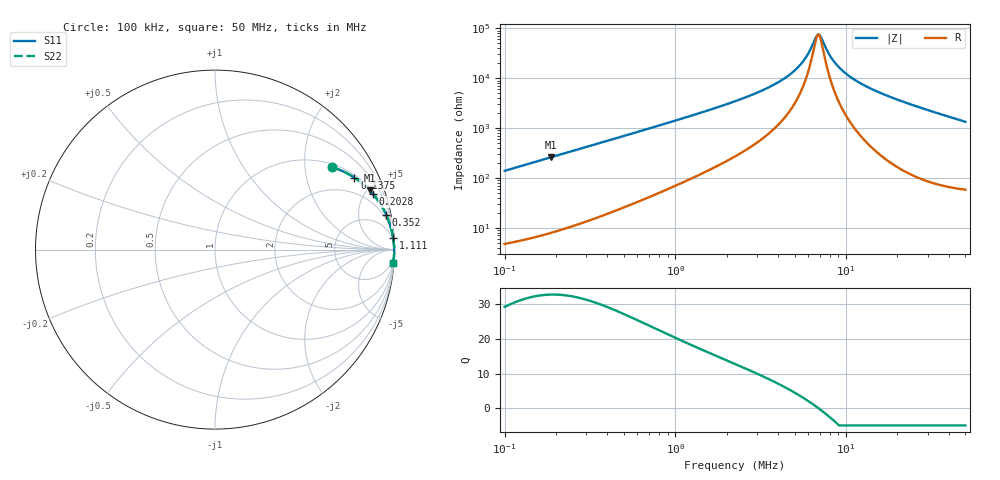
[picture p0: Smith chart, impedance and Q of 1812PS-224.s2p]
# MHz S MA R 50
!Freq  MagS11  AngS11  MagS21  AngS21  MagS12  AngS12  MagS22  AngS22
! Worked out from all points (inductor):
!   801 points, 100 kHz to 50 MHz, reference 50 ohm
!   read as one part in series: L = 220 uH near 103.2 kHz
!   highest Q = 32.8 at 186.2 kHz (marker M1), where L = 220 uH
!   self-resonance near 6.844 MHz
!   S11 on the Smith chart (normalised r, x): 100 kHz: 1.09, +2.76; 137.5 kHz: 1.12, +3.80; 202.8 kHz: 1.17, +5.61; 352 kHz: 1.32, +9.75; 1.111 MHz: 3, +31; 50 MHz: 2, -27
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0.1  0.7976 35.2  0.5766 -52.9  0.5766 -52.9  0.7976 35.2
0.1375062  0.8739 27.3  0.4595 -60.9  0.4595 -60.9  0.8739 27.3
0.1861646  0.9228 21.0  0.3583 -67.3  0.3583 -67.3  0.9228 21.0
0.2027719  0.933 19.4  0.3326 -68.8  0.3326 -68.8  0.933 19.4
0.2831897  0.9617 14.2  0.2453 -74.0  0.2453 -74.0  0.9617 14.2
0.351999  0.9733 11.5  0.1996 -76.6  0.1996 -76.6  0.9733 11.5
0.7957584  0.9921 5.1  0.08906 -82.4  0.08906 -82.4  0.9921 5.1
1.11135  0.9947 3.6  0.06314 -83.4  0.06314 -83.4  0.9947 3.6
2.236068  0.9973 1.7  0.02895 -83.9  0.02895 -83.9  0.9973 1.7
3.401461  0.998 0.9  0.01615 -82.6  0.01615 -82.6  0.998 0.9
4.534118  0.9984 0.5  0.009156 -79.5  0.009156 -79.5  0.9984 0.5
5.505993  0.9985 0.3  0.004944 -72.6  0.004944 -72.6  0.9985 0.3
5.950765  0.9986 0.2  0.003374 -65.2  0.003374 -65.2  0.9986 0.2
6.332315  0.9986 0.1  0.002225 -51.9  0.002225 -51.9  0.9986 0.1
6.686186  0.9987 0.0  0.001471 -24.5  0.001471 -24.5  0.9987 0.0
6.950996  0.9987 -0.0  0.001333 8.8  0.001333 8.8  0.9987 -0.0
7.170375  0.9987 -0.0  0.001558 33.3  0.001558 33.3  0.9987 -0.0
8.246482  0.9988 -0.2  0.004008 71.8  0.004008 71.8  0.9988 -0.2
9.632587  0.9988 -0.4  0.007283 80.3  0.007283 80.3  0.9988 -0.4
12.35099  0.9988 -0.7  0.01303 84.3  0.01303 84.3  0.9988 -0.7
17.7937  0.9986 -1.3  0.02309 85.9  0.02309 85.9  0.9986 -1.3
50  0.994 -4.3  0.07441 83.3  0.07441 83.3  0.994 -4.3
